FUNCTION_BLOCK FB_MEM_TO_DATA_ST_EL5131_CamData
VAR_INPUT
	nNo			:	UDINT;
	nStartAdr	:	UDINT;
END_VAR
VAR_OUTPUT
END_VAR
VAR
END_VAR

//	//_bVaild := pstEL5131_CamData;
//	MEMCPY(ADR(_bVaild),(pstEL5131_CamData+16*(cNum-1)),1);
//	//_bOutputState := pstEL5131_CamData+1;
//	MEMCPY(ADR(_bOutputState),pstEL5131_CamData+16*(cNum-1)+1,1);
//	//_bBackward := pstEL5131_CamData+2;
//	MEMCPY(ADR(_bBackward),pstEL5131_CamData+16*(cNum-1)+2,1);
//	//_rPos := pstEL5131_CamData+8;
//	MEMCPY(ADR(_rPos),pstEL5131_CamData+16*(cNum-1)+8,1);

METHOD get_bBackward : BOOL
VAR_INPUT
	nNo			:	UDINT;
	nStartAdr	:	UDINT;
END_VAR

IF nNo =0 OR nStartAdr = 0
THEN 
	IF THIS^.nStartAdr <> 0 AND THIS^.nNo > 0
	THEN 
		MEMCPY(ADR(get_bBackward),THIS^.nStartAdr+16*(THIS^.nNo-1)+2,1);
	END_IF
	
ELSE
	MEMCPY(ADR(get_bBackward),nStartAdr+16*(nNo-1)+2,1);
END_IF
END_METHOD

METHOD get_bOutputState : BOOL
VAR_INPUT
	nNo			:	UDINT;
	nStartAdr	:	UDINT;
END_VAR

IF nNo =0 OR nStartAdr = 0
THEN 
	IF THIS^.nStartAdr <> 0 AND THIS^.nNo > 0
	THEN 
		MEMCPY(ADR(get_bOutputState),THIS^.nStartAdr+16*(THIS^.nNo-1)+1,1);
	END_IF
	
ELSE
	MEMCPY(ADR(get_bOutputState),nStartAdr+16*(nNo-1)+1,1);
END_IF
END_METHOD

METHOD get_bVaild : BOOL
VAR_INPUT
	nNo			:	UDINT;
	nStartAdr	:	UDINT;
END_VAR

IF nNo =0 OR nStartAdr = 0
THEN 
	IF THIS^.nStartAdr <> 0 AND THIS^.nNo > 0
	THEN 
		MEMCPY(ADR(get_bVaild),THIS^.nStartAdr+16*(THIS^.nNo-1),1);
	END_IF
	
ELSE
	MEMCPY(ADR(get_bVaild),nStartAdr+16*(nNo-1),1);
END_IF
END_METHOD

METHOD get_nDuration : UDINT
VAR_INPUT
	nNo			:	UDINT;
	nStartAdr	:	UDINT;
END_VAR
IF nNo =0 OR nStartAdr = 0
THEN 
	IF THIS^.nStartAdr <> 0 AND THIS^.nNo > 0
	THEN 
		MEMCPY(ADR(get_nDuration),THIS^.nStartAdr+16*(THIS^.nNo-1)+4,1);
	END_IF
	
ELSE
	MEMCPY(ADR(get_nDuration),nStartAdr+16*(nNo-1)+4,4);
END_IF
END_METHOD

METHOD get_rPos : LREAL
VAR_INPUT
	nNo			:	UDINT;
	nStartAdr	:	UDINT;
END_VAR
IF nNo = 0 OR nStartAdr = 0
THEN 
	IF THIS^.nStartAdr <> 0 AND THIS^.nNo > 0
	THEN 
		MEMCPY(ADR(get_rPos),THIS^.nStartAdr+16*(THIS^.nNo-1)+8,8);
	END_IF
	
ELSE
	MEMCPY(ADR(get_rPos),nStartAdr+16*(nNo-1)+8,8);
END_IF
END_METHOD

END_FUNCTION_BLOCK
